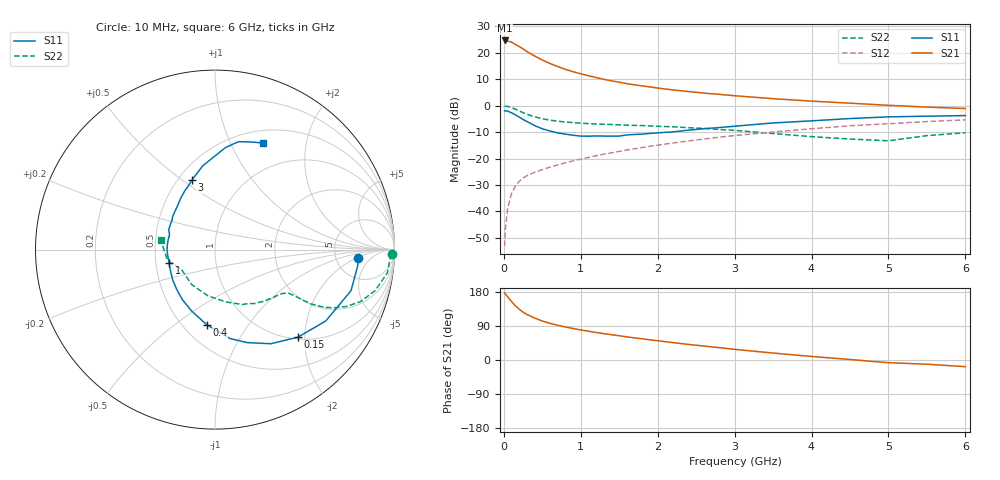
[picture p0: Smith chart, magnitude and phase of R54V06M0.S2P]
! SIEMENS Small Signal Semiconductors
! BFR183
! Si NPN RF Bipolar Junction Transistor in SOT23
! VCE = 4 V  IC = 6 mA
! Common Emitter S-Parameters:  May  1996
# GHz  S  MA  R  50
!  f  S11  S21  S12  S22
! GHz  MAG  ANG  MAG  ANG  MAG  ANG  MAG  ANG
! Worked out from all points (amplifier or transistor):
!   36 points, 10 MHz to 6 GHz, reference 50 ohm
!   highest |S21| = 24.7 dB at 10 MHz (marker M1)
!   |S21| within 3 dB of that: start of sweep to 238.1 MHz
!   unconditionally stable (mu >= 1): 962 MHz to 2.602 GHz
!   at 250 MHz: K = 0.47, MSG = 24.4 dB, |S12| = -27.4 dB
!   at 1.4 GHz: K = 1.06, MAG = 12.1 dB, |S12| = -17.8 dB
!   at 6 GHz: K = 0.88, MSG = 2.1 dB, |S12| = -5.3 dB
!   lowest NFmin = 1.20 dB at 450 MHz
!   S11 on the Smith chart (normalised r, x): 10 MHz: 8.41, -2.29; 150 MHz: 1.04, -1.85; 400 MHz: 0.65, -0.66; 1 GHz: 0.59, -0.09; 3 GHz: 0.58, +0.55; 6 GHz: 0.65, +1.33
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0.01  0.8009 -3.5  17.17 177.3  0.0022 88.4  0.9867 -1.5
0.02  0.7999 -6.7  16.89 174.3  0.0047 89.9  0.9761 -3.0
0.05  0.7917 -16.8  16.8 166.6  0.0114 81.7  0.9696 -7.6
0.1  0.7342 -32.8  15.96 154.4  0.0218 73.5  0.9207 -14.4
0.15  0.6722 -46.5  14.47 142.9  0.0303 67.7  0.8604 -19.7
0.2  0.61 -59.3  13.18 134.0  0.0369 64.4  0.798 -23.4
0.25  0.5487 -70.8  11.85 126.2  0.0429 60.7  0.7374 -26.1
0.3  0.5031 -80.3  10.6 120.1  0.0474 59.7  0.6897 -27.8
0.4  0.4214 -96.2  8.735 110.8  0.0551 57.9  0.6194 -29.4
0.5  0.3657 -111.0  7.311 102.8  0.0619 57.7  0.5666 -29.9
0.6  0.3321 -123.4  6.295 96.8  0.069 57.9  0.5324 -30.0
0.8  0.2897 -144.5  4.88 87.2  0.0831 58.7  0.4922 -30.4
1  0.266 -164.3  4.009 79.3  0.0976 60.0  0.4679 -31.2
1.1  0.2652 -171.9  3.693 76.0  0.1053 60.6  0.4591 -32.1
1.3  0.2666 174.0  3.163 69.6  0.1211 60.8  0.4447 -33.5
1.6  0.2805 156.8  2.612 60.9  0.1453 60.3  0.4283 -37.0
2.2  0.3202 130.9  1.985 45.9  0.197 57.5  0.3995 -46.0
3  0.4093 108.2  1.545 28.1  0.2724 50.7  0.3422 -63.4
3.5  0.472 98.3  1.359 18.3  0.3182 45.1  0.2974 -78.5
4.5  0.5718 84.1  1.117 1.3  0.4173 33.2  0.2343 -123.7
5.5  0.6336 71.1  0.941 -11.1  0.5013 20.9  0.2718 -166.8
6  0.6509 65.8  0.885 -17.6  0.5403 12.9  0.3077 169.6
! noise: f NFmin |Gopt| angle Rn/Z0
0.45  1.2  0.21  41  0.24
0.9  1.25  0.24  101  0.21
1.8  2  0.32  175  0.14
